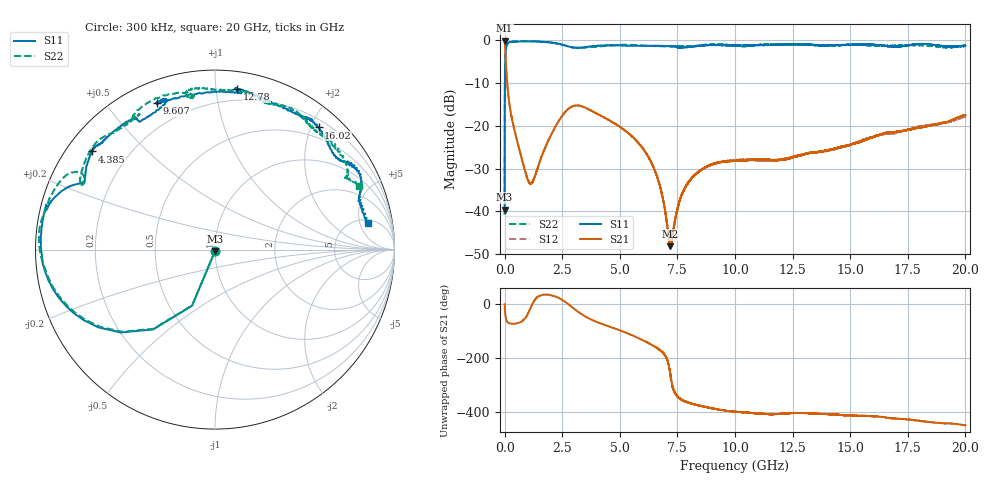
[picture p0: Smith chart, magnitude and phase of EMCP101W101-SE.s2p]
!EMCP101W101
!Johanson Technology Inc.
!www.johansontechnology.com
!Test Board Conditions:
!Substrate Type  RO4350B
!Substrate Thickness  10 mil
!Substrate Dk  3.66
!TL Type: GCPW
!TL Trace Width  20 mil
!TL Gap  10 mil
!PART MODE SINGLE ENDED (AKA BYPASS)
!DUT TOPOLOGY	SERIES-SHUNT
# MHz S  dB  R 50
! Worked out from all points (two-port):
!   20001 points, 300 kHz to 20 GHz, reference 50 ohm
!   highest |S21| = -0.02 dB at 1.3 MHz (marker M1); lowest = -48.1 dB at 7.178 GHz (marker M2)
!   |S21| within 3 dB of the highest: start of sweep to 34.9 MHz
!   lowest |S11| = -39.5 dB at 300 kHz (marker M3), VSWR 1.02, Z = 49.9 - j1.05 ohm
!   |S11| at or under -10 dB: start of sweep to 12.31 MHz
!   |S22| runs from -40.7 to -0.1 dB; largest |S21 - S12| = 0.0077
!   S11 on the Smith chart (normalised r, x): 300 kHz: 1.00, -0.02; 4.385 GHz: 0.07, +0.35; 9.607 GHz: 0.09, +0.68; 12.78 GHz: 0.12, +1.14; 16.02 GHz: 0.32, +2.12; 20 GHz: 5.69, +6.64
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0.3  -39.54 -93.8  -0.02 -0.3  -0.00 -0.5  -40.74 -92.2
1.3  -28.70 -92.8  -0.02 -2.1  -0.01 -2.0  -28.78 -93.1
101.298  -0.93 -161.0  -9.27 -63.9  -9.22 -63.9  -1.01 -160.8
129.298  -0.70 -165.2  -11.07 -66.9  -11.03 -67.1  -0.79 -164.8
419.294  -0.28 -179.6  -20.79 -72.6  -20.77 -72.8  -0.27 -178.0
1097.284  -0.23 169.4  -33.38 -20.2  -33.45 -20.0  -0.16 171.3
2433.264  -0.91 157.9  -18.15 19.1  -18.13 18.7  -0.89 151.6
3334.25  -1.66 151.3  -15.38 -37.0  -15.39 -37.0  -1.73 153.5
4385.234  -1.14 141.4  -18.21 -78.2  -18.20 -78.2  -1.29 149.5
5871.212  -1.24 133.1  -24.35 -128.4  -24.33 -127.9  -1.16 133.1
6667.2  -1.26 124.8  -32.74 -165.3  -32.62 -166.1  -1.34 128.2
7178.192  -1.33 121.5  -48.11 106.8  -47.67 108.4  -1.35 124.9
7610.186  -1.64 118.7  -37.30 9.7  -37.21 9.7  -1.27 119.7
7983.18  -1.49 112.9  -33.15 -5.3  -33.15 -4.8  -1.31 121.5
9607.156  -1.13 111.6  -28.28 -34.7  -28.24 -33.8  -1.00 101.8
10000.15  -1.19 109.1  -28.18 -38.5  -28.01 -38.2  -1.21 98.1
11342.13  -1.06 82.0  -27.90 -47.0  -28.03 -47.1  -0.90 98.9
12780.11  -0.89 82.2  -27.01 -43.9  -26.88 -43.7  -1.00 82.3
13334.1  -1.03 75.4  -26.22 -45.4  -26.17 -45.6  -1.06 75.4
16017.06  -0.99 49.7  -22.59 -55.6  -22.45 -57.1  -1.18 53.6
16667.05  -1.38 40.9  -21.48 -61.7  -21.74 -61.9  -1.22 50.7
20000  -1.28 10.0  -17.43 -89.6  -17.76 -87.6  -1.08 24.0
